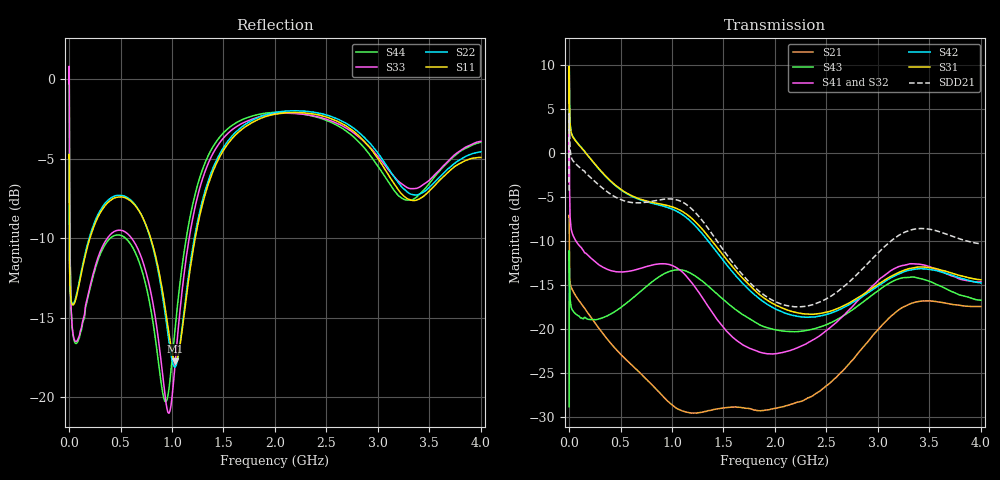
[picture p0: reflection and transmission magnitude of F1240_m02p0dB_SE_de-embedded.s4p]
! Integrated Device Technology
! Corporate Headquarters
! 6024 Silver Creek Valley Road
! San Jose, CA 95138  USA
! Phone:  1-408-284-8200
! Toll Free:  1-800-223-1366
! Webpage:  http://www.idt.com/
! Timing and RF Division
! 515 Groton Road, Suite 102
! Westford, MA 01886-6024
! Device:  F1240
! Description: Dual Intermediate Frequency Digital Variable Gain Amplifier
! Frequency:  10.0 -  500.00 MHz
! Package:  5x5 mm QFN Plastic Package: 32 pin
! Ports:  8 RF, 20 DC
!  Pin  1  = GA3 / Data  Pin 17  = RF OUT_B+
!  Pin  2  = GA4 / CLK  Pin 18  = RF OUT_B-
!  Pin  3  = GA5  Pin 19  = STBY_B
!  Pin  4  = VMODE  Pin 20  = Ground
!  Pin  5  = No Connect  Pin 21  = Ground
!  Pin  6  = GB5  Pin 22  = STB_A
!  Pin  7  = GB4  Pin 23  = RF OUT_A-  = Port 4
!  Pin  8  = GB3  Pin 24  = RF OUT_A+  = Port 3
!  Pin  9  = GB2  Pin 25  = GA0
!  Pin 10  = GB1  Pin 26  = ISET_A
!  Pin 11  = RF IN_B+  Pin 27  = VCC
!  Pin 12  = RF IN_B-  Pin 28  = Ground
!  Pin 13  = Ground  Pin 29  = RF IN_A-  = Port 2
!  Pin 14  = VCC  Pin 30  = RF IN_A+  = Port 1
!  Pin 15  = ISET_B  Pin 31  = GA1
!  Pin 16  = GB0  Pin 32  = GA2 / CSb
! Gain  = +19.5 dB
! State  = 1
! Voltage  = +5.00 V
! Current  = 85.292 mA (one channel only)
! Temperture  =  +25 C
! Test Date  =  2017-10-18
! Board  =  EB4031
! Data:  The device was measured on a custom evaluation board which has
!  individual transmission lines to the RF pins.  Data was collected
!  using a calibrated network analyzer.  The evaluation board was
!  de-embedded using Automatic Fixture Removal.
!  The reference plane is the edge of the package pin.
!  Only Channel A was measured.
!  This data is in single-ended operation.  If your needs are balanced
!  or differential S-parameters then this file needs to be used a
!  linear simulator.
! File Date:  2017-11-10  MJV
! Note:
!  Integrated Device Technology supplies this data as a sample of measured
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# Hz S dB R 100
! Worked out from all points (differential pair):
!   410 points, 500 kHz to 4 GHz, reference 100 ohm
!   strongest paths, dB at 500 kHz, 930 MHz, 1.96 GHz, 2.98 GHz, 4 GHz:
!     S31: 2.3, -5.9, -17.0, -15.0, -14.4
!     S42: 2.3, -6.1, -17.4, -15.2, -14.7
!     S41: -3.3, -12.6, -22.8, -14.7, -14.6
!     S32: -3.2, -12.7, -22.8, -15.1, -15.1
!     S43: -28.8, -13.7, -19.9, -15.8, -16.7
!     S21: -7.2, -27.9, -29.1, -20.3, -17.4
!   taken as a pair (ports 1,2 in; 3,4 out), SDD21 dB: -4.2, -5.2, -16.6, -11.6, -10.3
!   lowest |S11| = -17.7 dB at 1.03 GHz (marker M1), VSWR 1.30, Z = 78.2 - j7.66 ohm
!   |S11| at or under -10 dB: 3.388 MHz to 202.9 MHz (199.5 MHz wide, 193 % of centre); 792.6 MHz to 1.225 GHz (432.7 MHz wide, 42.9 % of centre)
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500000  -4.98 -5.6  -7.24 -5.8  -30.39 80.3  -36.31 78.2
        -7.24 -5.8  -4.98 -5.6  -36.28 77.3  -30.39 81.3
        2.29 -108.1  -3.23 -110.2  -0.27 0.6  -28.82 -41.7
        -3.26 -109.1  2.29 -107.0  -28.80 -41.7  -0.28 2.9
2000000  -6.83 -35.8  -9.72 -36.3  -20.95 30.0  -27.64 8.7
         -9.72 -36.3  -6.80 -35.9  -27.59 8.5  -20.94 30.3
         9.72 -175.3  3.64 166.7  -0.07 -48.2  -11.05 -136.8
         3.60 166.9  9.73 -175.0  -11.04 -136.8  -0.12 -47.9
4000000  -10.85 -36.9  -13.64 -27.6  -21.11 9.7  -30.78 -14.4
         -13.65 -27.6  -10.83 -37.2  -30.75 -14.7  -21.10 9.9
         6.61 160.9  -2.27 139.3  -4.54 -80.8  -13.19 178.3
         -2.32 139.4  6.61 161.1  -13.17 178.2  -4.59 -80.8
1.7e8  -10.77 -102.6  -17.93 -54.6  -23.45 -43.7  -35.66 -32.1
       -17.94 -54.5  -10.61 -104.0  -35.73 -31.7  -23.47 -43.9
       -0.07 116.6  -11.46 88.7  -13.98 -145.2  -18.84 110.1
       -11.43 88.6  -0.07 115.7  -18.81 109.7  -14.11 -145.2
1.03e9  -17.74 -158.2  -29.28 175.2  -23.69 150.3  -31.60 -167.6
        -28.86 174.2  -18.11 -154.8  -31.57 -162.4  -24.38 149.5
        -6.20 -92.5  -13.10 173.6  -17.92 -113.1  -13.45 -125.4
        -12.91 169.6  -6.49 -95.2  -13.27 -125.3  -15.68 -107.9
2.86e9  -3.87 97.4  -22.05 -27.9  -25.35 -151.9  -27.61 -135.9
        -21.99 -27.8  -3.61 98.4  -28.40 -123.7  -26.55 -146.4
        -16.02 -63.8  -16.49 -149.4  -3.89 102.1  -17.75 -81.9
        -16.12 -159.9  -16.20 -60.7  -16.87 -79.3  -4.27 95.1
4e9  -4.93 -141.5  -17.44 106.0  -23.74 -38.6  -24.81 -23.0
     -17.41 105.9  -4.57 -139.7  -25.76 -7.8  -25.45 -31.7
     -14.38 46.3  -15.09 -57.3  -3.91 -133.8  -18.33 65.9
     -14.61 -70.5  -14.74 52.2  -16.70 57.7  -3.97 -143.7
